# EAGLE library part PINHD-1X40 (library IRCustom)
Pinouts for OLED/LCD displays with flex ribbons
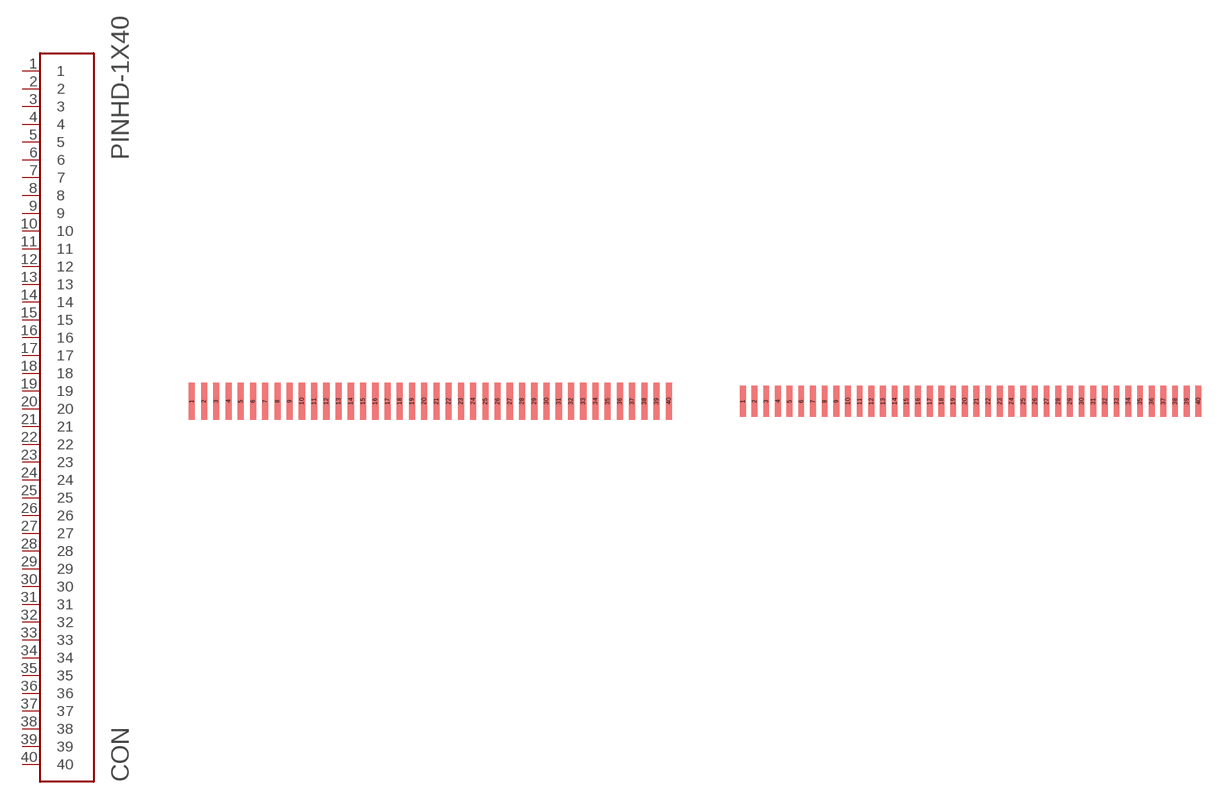
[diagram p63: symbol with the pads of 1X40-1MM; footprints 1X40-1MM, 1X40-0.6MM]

Designator prefix CON

## PINHD-1X40-1MM  [1X40-1MM]
1  1
2  2
3  3
4  4
5  5
6  6
7  7
8  8
9  9
10  10
11  11
12  12
13  13
14  14
15  15
16  16
17  17
18  18
19  19
20  20
21  21
22  22
23  23
24  24
25  25
26  26
27  27
28  28
29  29
30  30
31  31
32  32
33  33
34  34
35  35
36  36
37  37
38  38
39  39
40  40

## PINHD-1X40-0.6MM  [1X40-0.6MM]
Pads as for 1X40-1MM

## PINHD-1X40-0.7MM  [1X40-0.7MM]
Pads as for 1X40-1MM

## PINHD-1X40-0.8MM  [1X40-0.8MM]
Pads as for 1X40-1MM

## PINHD-1X40-0.5MM  [1X40-0.5MM]
Pads as for 1X40-1MM

## Footprint 1X40-1MM (pad centres in mm)
smd 0.5 x 3: 1 -19.5,-0.17; 2 -18.5,-0.17; 3 -17.5,-0.17; 4 -16.5,-0.17; 5 -15.5,-0.17; 6 -14.5,-0.17; 7 -13.5,-0.17; 8 -12.5,-0.17; 9 -11.5,-0.17; 10 -10.5,-0.17; 11 -9.5,-0.17; 12 -8.5,-0.17; 13 -7.5,-0.17; 14 -6.5,-0.17; 15 -5.5,-0.17; 16 -4.5,-0.17; 17 -3.5,-0.17; 18 -2.5,-0.17; 19 -1.5,-0.17; 20 -0.5,-0.17; 21 0.5,-0.17; 22 1.5,-0.17; 23 2.5,-0.17; 24 3.5,-0.17; 25 4.5,-0.17; 26 5.5,-0.17; 27 6.5,-0.17; 28 7.5,-0.17; 29 8.5,-0.17; 30 9.5,-0.17; 31 10.5,-0.17; 32 11.5,-0.17; 33 12.5,-0.17; 34 13.5,-0.17; 35 14.5,-0.17; 36 15.5,-0.17; 37 16.5,-0.17; 38 17.5,-0.17; 39 18.5,-0.17; 40 19.5,-0.17

## Footprint 1X40-0.6MM (pad centres in mm)
smd 0.3 x 1.6: 1 -11.7,0; 2 -11.1,0; 3 -10.5,0; 4 -9.9,0; 5 -9.3,0; 6 -8.7,0; 7 -8.1,0; 8 -7.5,0; 9 -6.9,0; 10 -6.3,0; 11 -5.7,0; 12 -5.1,0; 13 -4.5,0; 14 -3.9,0; 15 -3.3,0; 16 -2.7,0; 17 -2.1,0; 18 -1.5,0; 19 -0.9,0; 20 -0.3,0; 21 0.3,0; 22 0.9,0; 23 1.5,0; 24 2.1,0; 25 2.7,0; 26 3.3,0; 27 3.9,0; 28 4.5,0; 29 5.1,0; 30 5.7,0; 31 6.3,0; 32 6.9,0; 33 7.5,0; 34 8.1,0; 35 8.7,0; 36 9.3,0; 37 9.9,0; 38 10.5,0; 39 11.1,0; 40 11.7,0

## Footprint 1X40-0.7MM (pad centres in mm)
smd 0.35 x 1.6: 1 -13.65,0; 2 -12.95,0; 3 -12.25,0; 4 -11.55,0; 5 -10.85,0; 6 -10.15,0; 7 -9.45,0; 8 -8.75,0; 9 -8.05,0; 10 -7.35,0; 11 -6.65,0; 12 -5.95,0; 13 -5.25,0; 14 -4.55,0; 15 -3.85,0; 16 -3.15,0; 17 -2.45,0; 18 -1.75,0; 19 -1.05,0; 20 -0.35,0; 21 0.35,0; 22 1.05,0; 23 1.75,0; 24 2.45,0; 25 3.15,0; 26 3.85,0; 27 4.55,0; 28 5.25,0; 29 5.95,0; 30 6.65,0; 31 7.35,0; 32 8.05,0; 33 8.75,0; 34 9.45,0; 35 10.15,0; 36 10.85,0; 37 11.55,0; 38 12.25,0; 39 12.95,0; 40 13.65,0

## Footprint 1X40-0.8MM (pad centres in mm)
smd 0.4 x 2: 1 -15.6,0; 2 -14.8,0; 3 -14,0; 4 -13.2,0; 5 -12.4,0; 6 -11.6,0; 7 -10.8,0; 8 -10,0; 9 -9.2,0; 10 -8.4,0; 11 -7.6,0; 12 -6.8,0; 13 -6,0; 14 -5.2,0; 15 -4.4,0; 16 -3.6,0; 17 -2.8,0; 18 -2,0; 19 -1.2,0; 20 -0.4,0; 21 0.4,0; 22 1.2,0; 23 2,0; 24 2.8,0; 25 3.6,0; 26 4.4,0; 27 5.2,0; 28 6,0; 29 6.8,0; 30 7.6,0; 31 8.4,0; 32 9.2,0; 33 10,0; 34 10.8,0; 35 11.6,0; 36 12.4,0; 37 13.2,0; 38 14,0; 39 14.8,0; 40 15.6,0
